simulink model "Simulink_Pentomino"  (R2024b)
settings: Solver=FixedStepAuto  StartTime=0.0  StopTime=Inf  FixedStep=0.001  RelTol=1e-3  EnableMultiTasking=on
libraries: arduinolib x9

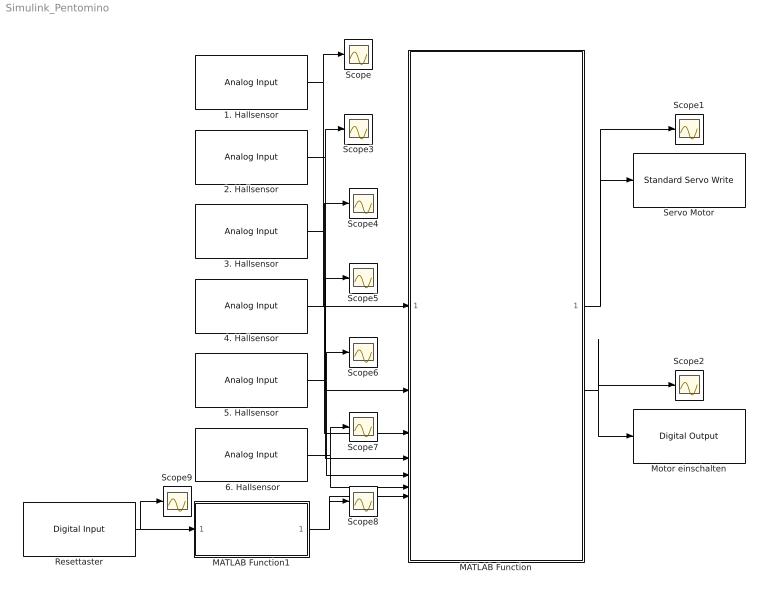
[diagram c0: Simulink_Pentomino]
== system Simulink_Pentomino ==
  " 6. Hallsensor" : arduinolib/Analog Input  pinNumber=5  ReadResultsOnly=off  ConversionTriggerSource=Software  ExternalTriggerType=uint32( 0 )  OutputDataType=uint16  EnableConversionCompleteNotify=off  EnableOuputStatus=off  SampleTime=Inf  blockPlatform=arduino
  1. Hallsensor : arduinolib/Analog Input  pinNumber=0  ReadResultsOnly=off  ConversionTriggerSource=Software  ExternalTriggerType=uint32( 0 )  OutputDataType=uint16  EnableConversionCompleteNotify=off  EnableOuputStatus=off  SampleTime=Inf  blockPlatform=arduino
  2. Hallsensor : arduinolib/Analog Input  pinNumber=1  ReadResultsOnly=off  ConversionTriggerSource=Software  ExternalTriggerType=uint32( 0 )  OutputDataType=uint16  EnableConversionCompleteNotify=off  EnableOuputStatus=off  SampleTime=Inf  blockPlatform=arduino
  3. Hallsensor : arduinolib/Analog Input  pinNumber=2  ReadResultsOnly=off  ConversionTriggerSource=Software  ExternalTriggerType=uint32( 0 )  OutputDataType=uint16  EnableConversionCompleteNotify=off  EnableOuputStatus=off  SampleTime=Inf  blockPlatform=arduino
  4. Hallsensor : arduinolib/Analog Input  pinNumber=3  ReadResultsOnly=off  ConversionTriggerSource=Software  ExternalTriggerType=uint32( 0 )  OutputDataType=uint16  EnableConversionCompleteNotify=off  EnableOuputStatus=off  SampleTime=Inf  blockPlatform=arduino
  5. Hallsensor : arduinolib/Analog Input  pinNumber=4  ReadResultsOnly=off  ConversionTriggerSource=Software  ExternalTriggerType=uint32( 0 )  OutputDataType=uint16  EnableConversionCompleteNotify=off  EnableOuputStatus=off  SampleTime=Inf  blockPlatform=arduino
  MATLAB Function : MATLAB Function  TreatAsAtomicUnit=on
  MATLAB Function1 : MATLAB Function  TreatAsAtomicUnit=on
  Motor einschalten : arduinolib/Digital Output  pinNumber=4  Direction=output  blockPlatform=arduino
  Resettaster : arduinolib/Digital Input  pinNumber=2  mode=Input Pullup  Direction=input  SampleTime=Inf  blockPlatform=arduino
  Scope{,1..9} (10 alike) : Scope
  Servo Motor : arduinolib/Standard Servo Write  pinNumber=3  ServoIndex=0  blockPlatform=ARDUINO
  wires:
  1. Hallsensor/1 -> Scope/1, MATLAB Function/1(A0)
  2. Hallsensor/1 -> Scope3/1, MATLAB Function/2(A1)
  3. Hallsensor/1 -> MATLAB Function/3(A2), Scope4/1
  4. Hallsensor/1 -> Scope5/1, MATLAB Function/4(A3)
  5. Hallsensor/1 -> Scope6/1, MATLAB Function/5(A4)
  " 6. Hallsensor"/1 -> Scope7/1, MATLAB Function/6(A5)
  MATLAB Function/2(MotorON) -> Motor einschalten/1, Scope2/1
  MATLAB Function/1(Drehwinkel) -> Servo Motor/1, Scope1/1
  MATLAB Function1/1(Taster) -> Scope8/1, MATLAB Function/7(Taster)
  Resettaster/1 -> MATLAB Function1/1(T), Scope9/1

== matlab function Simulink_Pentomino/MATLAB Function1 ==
function Taster = Entprellroutine(T)
    % Definition der Variablen
    persistent buttonState;  % Speichert den Zustand des Tasters
    persistent holdState;    % Speichert, ob der Taster gehalten wird
    if isempty(buttonState)
        buttonState = uint8(0);  % Initialisiere mit 0
    end
    if isempty(holdState)
        holdState = false;  % Initialisiere mit false
    end
    Taster=0;

    %Übergabe des Taster Inputs
    currentState = T;  

    % Die vorherigen Zustände in der 8-Bit-Variable speichern
    buttonState = bitshift(buttonState, 1) + uint8(currentState);

    % Steigende Flanke erkennen (Wechsel von 0 auf 1)
    if bitand(buttonState, uint8(3)) == uint8(1)
        Taster=1;
        holdState = true;  % Taster wird als gehalten markiert
    end

    % Fallende Flanke erkennen (Wechsel von 1 auf 0)
    if bitand(buttonState, uint8(3)) == uint8(2)
        Taster=0;
        holdState = false;  % Taster wird nicht mehr gehalten
    end

    % Erkennen, ob der Taster gehalten wird
    if holdState==true
        Taster=1;
    end
end

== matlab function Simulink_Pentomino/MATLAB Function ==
%*************************************************************** *
%                   Hochschule Hamm-Lippstadt                    *
%*************************************************************** *
% Modul	        :                                              *
%                                                                *
% Datum           : 07.01.2024                                   *
%                                                                *
% Funktion        : Ansteuerung der Motoren einer Geheimbox      *
%                                                                *
% Implementation  : MATLAB 2024b                                 *
%                                                                *
% Req. Toolbox    : -                                            *
%                                                                *
% Author          : Kevin Ernst, Timo Roch                       * 
%                                                                *
% Letzte Änderung : 07.01.2024                                   *
%*****************************************************************
function [Drehwinkel,MotorON] = Steuerung_Pentomino(A0,A1,A2,A3,A4,A5,Taster)
    persistent Init             % Initialiesierungs Variable
    persistent MotorNeutral     % Motor in einer Mittigen Stellung
    persistent MotorVorne       % Motor öffnet Klappe
    persistent MotorVerriegelt  % Motor verriegelt Klappe
    persistent Zustand          % Zustand des Programms
    
    persistent SchwelleHall     % Schaltschwelle der Hallsensoren
    persistent ZeitReturn       % Zeit die der Motor vorne bleibt befor er zurück in Neutral fährt => 10 = 1s
    persistent ZeitReturn_C     % Zählvariable für ZeitReturn
    persistent ZeitMotor        % Zeit die der Motor benötigt um zu fahren
    persistent ZeitMotor_C      % Zählvariable für ZeitMotor

    %Initialiesierung
    if isempty(Init)
        SchwelleHall=650;
        ZeitReturn=1000;
        ZeitReturn_C=ZeitReturn;
        MotorNeutral=129;
        MotorVorne=95;
        MotorVerriegelt=140;
        Zustand=5;
        Init = true;
        ZeitMotor=500;
        ZeitMotor_C=ZeitMotor;
    end

    % Setze Standardwerte für die Ausgaben
    Drehwinkel = MotorVerriegelt; % Standardwert, falls keine Bedingung erfüllt wird
    MotorON = 0;                  % Standardwert: Motor ist aus

    if (Init == true)

        % true=Alle 6 Hallsensoren in dem Durchlauf erkannt
        SechsMalHall = ((A0>=SchwelleHall)&&(A1>=SchwelleHall)&&(A2>=SchwelleHall)&&(A3>=SchwelleHall)&&(A4>=SchwelleHall)&&(A5>=SchwelleHall));

        switch Zustand
            case 0 %"Verriegelt"
                MotorON = 0;
                Drehwinkel = MotorVerriegelt;
                if ((SechsMalHall)&&(Taster==1))
                   Zustand=1; %"Bewegung von Verriegelt zu Vorne";
                end

            case 1 %"Bewegung von Verriegelt zu Vorne"
                MotorON = 1;
                Drehwinkel = MotorVorne;
                if(ZeitMotor_C<=0)
                    Zustand=2; %"Vorne";
                    ZeitMotor_C=ZeitMotor;
                else
                    ZeitMotor_C=ZeitMotor_C-1;
                end

            case 2 %"Vorne"
                MotorON = 0;
                Drehwinkel = MotorVorne;
                if(ZeitReturn_C<=0)
                    Zustand=3; %"Bewegung von Vorne zu Neutral";
                    ZeitReturn_C=ZeitReturn;
                else
                    ZeitReturn_C=ZeitReturn_C-1;
                end

            case 3 %"Bewegung von Vorne zu Neutral"
                MotorON = 1;
                Drehwinkel = MotorNeutral;
                if(ZeitMotor_C<=0)
                    Zustand=4; %"Neutral";
                    ZeitMotor_C=ZeitMotor;
                else
                    ZeitMotor_C=ZeitMotor_C-1;
                end

            case 4 %"Neutral"
                MotorON = 0;
                Drehwinkel = MotorNeutral;
                if ((~SechsMalHall)&&(Taster==0))
                   Zustand=5; %"Bewegung von neutral zu Verriegelt";
                end

            case 5 %"Bewegung von neutral zu Verriegelt"
                MotorON = 1;
                Drehwinkel = MotorVerriegelt;
                if(ZeitMotor_C<=0)
                    Zustand=0; %"Verriegelt";
                    ZeitMotor_C=ZeitMotor;
                else
                    ZeitMotor_C=ZeitMotor_C-1;
                end
        end
    end
end
